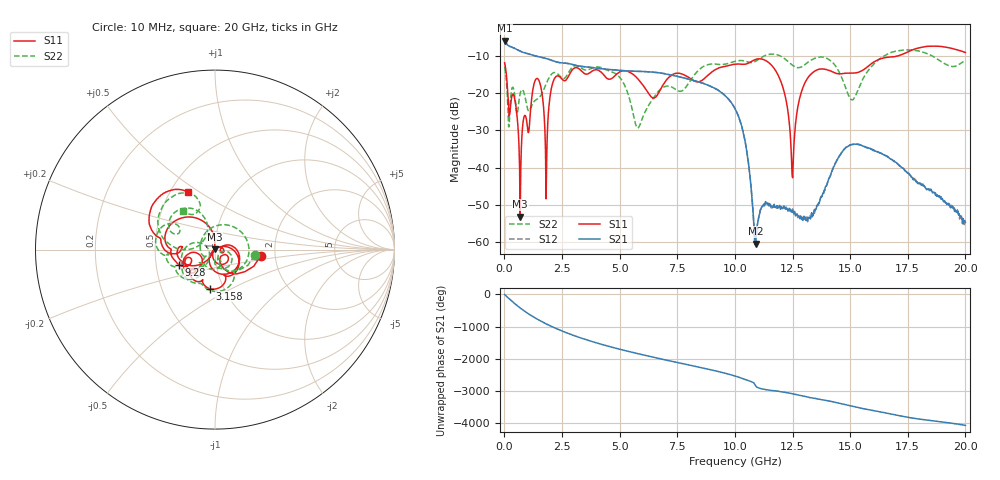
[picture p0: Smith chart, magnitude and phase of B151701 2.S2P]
!  2-Port S-parameters saved by WinCal
! VAR MeasName=S-Parameters (CALIBRATED_DATA) read from VNA (N5244A)
! VAR MeasDate=2015-12-24 19:08:28
! VAR NAME=B151701 2
! VAR FILENAME=B151701 2.S2P
! VAR DATE=2015-12-24 19:08:28
! VAR PHYS_PORTS=1,3
# Hz S DB R 50
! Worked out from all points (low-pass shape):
!   801 points, 10 MHz to 20 GHz, reference 50 ohm
!   highest |S21| = -5.85 dB at 10 MHz (marker M1); lowest = -60.4 dB at 10.9 GHz (marker M2)
!   |S21| within 3 dB of the highest: start of sweep to 739.7 MHz
!   lowest |S11| = -53.1 dB at 684.7 MHz (marker M3), VSWR 1.00, Z = 49.8 + j0.123 ohm
!   |S11| at or under -10 dB: start of sweep to 17.06 GHz
!   |S22| runs from -29.4 to -8.4 dB; largest |S21 - S12| = 0.0015
!   S11 on the Smith chart (normalised r, x): 10 MHz: 1.68, -0.12; 3.158 GHz: 0.86, -0.39; 9.28 GHz: 0.66, -0.12; 20 GHz: 0.61, +0.45
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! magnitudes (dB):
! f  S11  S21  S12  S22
! 10 MHz  -11.8  -5.9  -5.8  -13.0
! 209.9 MHz  -26.1  -7.3  -7.3  -29.0
! 459.8 MHz  -21.9  -8.0  -8.0  -21.1
! 684.7 MHz  -53.1  -8.7  -8.7  -20.1
! 1.359 GHz  -16.3  -10.0  -10.0  -21.8
! 1.809 GHz  -48.4  -10.7  -10.7  -17.5
! 2.159 GHz  -16.2  -11.4  -11.4  -14.4
! 3.158 GHz  -13.2  -12.6  -12.6  -12.7
! 3.358 GHz  -14.1  -12.8  -12.8  -13.4
! 4.958 GHz  -14.4  -13.8  -13.8  -15.4
! 5.782 GHz  -16.1  -14.1  -14.1  -29.4
! 6.682 GHz  -20.0  -14.5  -14.5  -19.5
! 9.28 GHz  -13.3  -19.2  -19.2  -12.2
! 10.01 GHz  -12.2  -24.1  -24.1  -11.4
! 10.48 GHz  -12.2  -34.2  -34.2  -11.4
! 10.9 GHz  -10.9  -60.4  -60.2  -11.4
! 11.98 GHz  -16.6  -51.2  -50.7  -10.0
! 12.5 GHz  -42.7  -51.9  -51.1  -12.5
! 13.35 GHz  -14.6  -53.2  -53.1  -11.0
! 15.1 GHz  -14.6  -33.7  -33.7  -21.8
! 16.68 GHz  -10.3  -37.2  -37.3  -9.3
! 20 GHz  -9.0  -54.7  -54.2  -11.1
